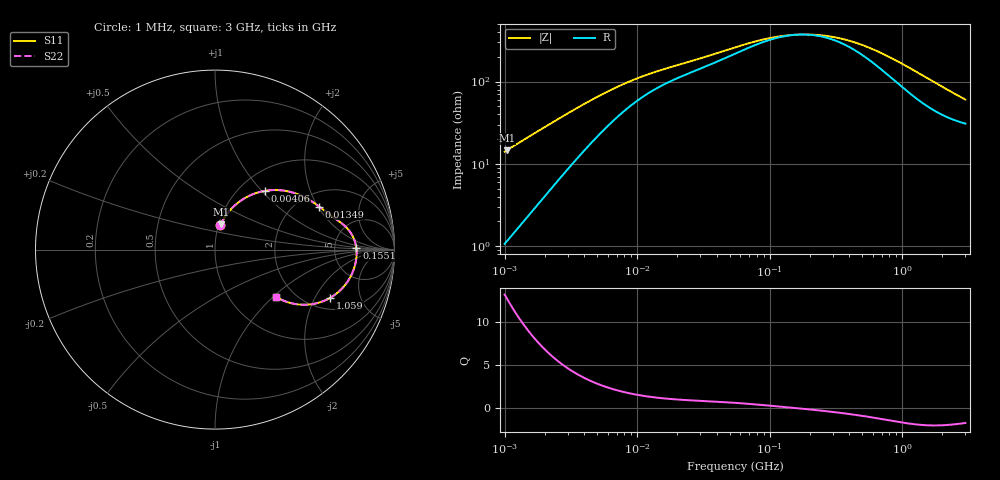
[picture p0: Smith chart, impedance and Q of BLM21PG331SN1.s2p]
! BLM21PG331SN1
# Hz S RI R 50
!Freq.(Hz) S11(Real) S11(Imag) S21(Real) S21(Imag) S12(Real) S12(Imag) S22(Real) S22(Imag)
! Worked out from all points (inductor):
!   401 points, 1 MHz to 3 GHz, reference 50 ohm
!   read as one part in series: L = 2.22 uH near 1.041 MHz
!   highest Q = 12.8 at 1.041 MHz (marker M1), where L = 2.23 uH
!   self-resonance near 167.6 MHz
!   S11 on the Smith chart (normalised r, x): 1 MHz: 1.02, +0.28; 4.06 MHz: 1.30, +1.04; 13.49 MHz: 2.59, +2.05; 155.1 MHz: 8.40, +0.37; 1.059 GHz: 2.59, -2.69; 3 GHz: 1.62, -1.04
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1000000  0.0292 0.1349  0.9708 -0.1349  0.9708 -0.1349  0.0292 0.1349
1040844  0.0315 0.1398  0.9685 -0.1398  0.9685 -0.1398  0.0315 0.1398
1492300  0.0611 0.1909  0.9389 -0.1909  0.9389 -0.1909  0.0611 0.1909
2055611  0.1064 0.2426  0.8936 -0.2426  0.8936 -0.2426  0.1064 0.2426
2775447  0.1701 0.2891  0.8299 -0.2891  0.8299 -0.2891  0.1701 0.2891
3823119  0.2599 0.3236  0.7401 -0.3236  0.7401 -0.3236  0.2599 0.3236
4059721  0.2785 0.3273  0.7215 -0.3273  0.7215 -0.3273  0.2785 0.3273
5481359  0.3731 0.3299  0.6269 -0.3299  0.6269 -0.3299  0.3731 0.3299
7703107  0.4699 0.3051  0.5301 -0.3051  0.5301 -0.3051  0.4699 0.3051
1.349163e7  0.5803 0.2396  0.4197 -0.2396  0.4197 -0.2396  0.5803 0.2396
1.461624e7  0.5918 0.2307  0.4082 -0.2307  0.4082 -0.2307  0.5918 0.2307
5.477226e7  0.7377 0.1171  0.2623 -0.1171  0.2623 -0.1171  0.7377 0.1171
9.787053e7  0.7752 0.0573  0.2248 -0.0573  0.2248 -0.0573  0.7752 0.0573
1.550909e8  0.7875 0.00837  0.2125 -0.00837  0.2125 -0.00837  0.7875 0.00837
2.094008e8  0.789 -0.0245  0.211 0.0245  0.211 0.0245  0.789 -0.0245
2.884452e8  0.7853 -0.0623  0.2147 0.0623  0.2147 0.0623  0.7853 -0.0623
3.894533e8  0.7755 -0.1025  0.2245 0.1025  0.2245 0.1025  0.7755 -0.1025
5.696638e8  0.7487 -0.1622  0.2513 0.1622  0.2513 0.1622  0.7487 -0.1622
8.005644e8  0.7027 -0.2218  0.2973 0.2218  0.2973 0.2218  0.7027 -0.2218
1.059487e9  0.6431 -0.2678  0.3569 0.2678  0.3569 0.2678  0.6431 -0.2678
1.747494e9  0.4939 -0.3074  0.5061 0.3074  0.5061 0.3074  0.4939 -0.3074
3e9  0.3398 -0.2625  0.6602 0.2625  0.6602 0.2625  0.3398 -0.2625
